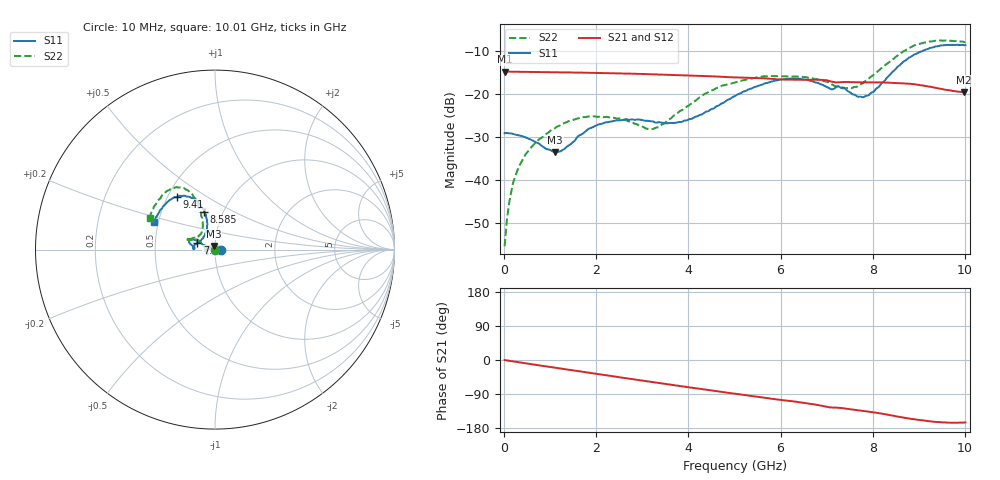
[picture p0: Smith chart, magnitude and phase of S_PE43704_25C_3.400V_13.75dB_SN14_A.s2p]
! Device ID: PE43704
! Dir: z:\PE43704\PE43704_Char_1_20130516\PE43704\AMB\3p400V\13p75dB
! Serial: 14
! Insertion: A
! Impedance: 50 ohm
! Temp: Amb
! VDD: 3.400V
! Attenuation Step: 13.75dB
! IDD: 1.140292e-01mA
#  Hz  S  RI  R  50
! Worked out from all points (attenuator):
!   401 points, 10 MHz to 10.01 GHz, reference 50 ohm
!   highest |S21| = -14.73 dB at 10 MHz (marker M1); lowest = -19.5 dB at 9.985 GHz (marker M2)
!   lowest |S11| = -33.4 dB at 1.11 GHz (marker M3), VSWR 1.04, Z = 49.4 + j2.02 ohm
!   |S11| at or under -10 dB: start of sweep to 9.069 GHz
!   |S22| runs from -55.3 to -7.5 dB; largest |S21 - S12| = 0.0013
!   S11 on the Smith chart (normalised r, x): 10 MHz: 1.07, +0.00; 7.51 GHz: 0.82, +0.06; 8.585 GHz: 0.82, +0.36; 9.41 GHz: 0.56, +0.38; 10.01 GHz: 0.47, +0.17
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1e7  0.0353 0.000259  0.1834 -0.000679  0.1835 -0.000689  0.00165 0.000446
1.6e8  0.0344 0.00614  0.1827 -0.00996  0.1827 -0.00986  0.00143 0.00743
3.35e8  0.0306 0.0126  0.1814 -0.0201  0.1814 -0.0201  -0.00178 0.0148
6.35e8  0.0196 0.0209  0.1778 -0.0373  0.1778 -0.0372  -0.0111 0.0232
1.11e9  -0.00601 0.0204  0.169 -0.0631  0.1691 -0.063  -0.0333 0.0233
1.685e9  -0.0342 0.00227  0.1531 -0.0915  0.1531 -0.0914  -0.0537 0.00538
2.41e9  -0.0449 -0.0208  0.1262 -0.1214  0.1264 -0.1213  -0.0517 -0.0111
3.11e9  -0.0424 -0.0249  0.0952 -0.1427  0.0953 -0.1426  -0.0396 -0.00122
3.36e9  -0.0427 -0.0204  0.083 -0.1481  0.0832 -0.1481  -0.0411 0.00697
4.035e9  -0.0514 0.00306  0.0495 -0.1574  0.0499 -0.1573  -0.0686 0.0324
4.46e9  -0.0619 0.0204  0.0285 -0.16  0.0288 -0.1602  -0.0948 0.0538
5.01e9  -0.0859 0.0413  0.00286 -0.1573  0.00298 -0.1573  -0.1257 0.055
5.96e9  -0.1354 0.0564  -0.0375 -0.1443  -0.0371 -0.1443  -0.1532 0.0522
6.685e9  -0.1385 0.032  -0.0655 -0.132  -0.0658 -0.1319  -0.1442 0.0525
7.51e9  -0.0976 0.0382  -0.0891 -0.1061  -0.0888 -0.1064  -0.0811 0.0849
7.86e9  -0.0629 0.0723  -0.0979 -0.0965  -0.098 -0.097  -0.0687 0.1266
8.36e9  -0.0447 0.1594  -0.1118 -0.0778  -0.1115 -0.0783  -0.0841 0.2214
8.585e9  -0.0596 0.2087  -0.1163 -0.0665  -0.1157 -0.0673  -0.1061 0.2723
8.935e9  -0.1058 0.2746  -0.1197 -0.0507  -0.1192 -0.0496  -0.1634 0.3361
9.41e9  -0.2114 0.2935  -0.1126 -0.0331  -0.1128 -0.0327  -0.2557 0.3316
9.985e9  -0.3326 0.1659  -0.102 -0.0273  -0.1023 -0.0274  -0.36 0.1848
1.001e10  -0.3378 0.1562  -0.1022 -0.0279  -0.1027 -0.028  -0.3641 0.1768
